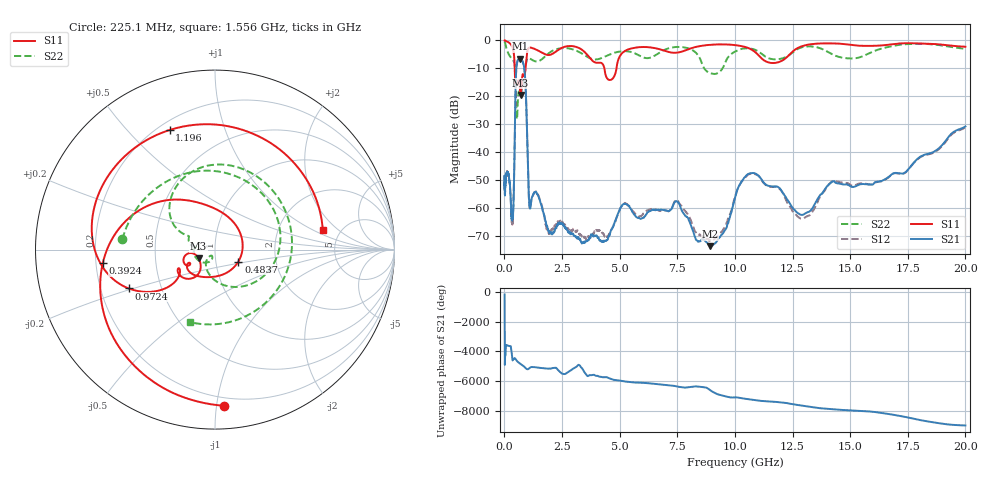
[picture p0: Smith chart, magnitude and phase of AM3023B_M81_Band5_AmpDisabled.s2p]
!Agilent Technologies,E8364B,MY43040894,A.07.50.67
!Agilent E8364B: A.07.50.67
!Date: Tuesday, October 27, 2020 10:38:44
!Correction: S11(Full 2 Port(1,2))
!S21(Full 2 Port(1,2))
!S12(Full 2 Port(1,2))
!S22(Full 2 Port(1,2))
!S2P File: Measurements: S11, S21, S12, S22:Log Frequency Sweep
# Hz S  dB  R 50
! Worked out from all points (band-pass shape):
!   3201 points, 10 MHz to 20 GHz, reference 50 ohm
!   highest |S21| = -6.78 dB at 689.1 MHz (marker M1); lowest = -73.7 dB at 8.919 GHz (marker M2)
!   |S21| within 3 dB of the highest: 523.8 MHz to 855.6 MHz (331.8 MHz wide, 48.1 % of centre)
!   lowest |S11| = -19.7 dB at 704 MHz (marker M3), VSWR 1.23, Z = 41.5 - j4.14 ohm
!   |S11| at or under -10 dB: 447.3 MHz to 919.4 MHz (472.2 MHz wide, 69.1 % of centre); 4.332 GHz to 4.868 GHz (536.3 MHz wide, 11.7 % of centre)
!   |S22| runs from -28.4 to -0.7 dB; largest |S21 - S12| = 0.007
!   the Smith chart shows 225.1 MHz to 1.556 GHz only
!   S11 on the Smith chart (normalised r, x): 225.1 MHz: 0.15, -1.05; 392.4 MHz: 0.23, -0.06; 483.7 MHz: 1.29, -0.17; 972.4 MHz: 0.32, -0.19; 1.196 GHz: 0.24, +0.66; 1.556 GHz: 3.65, +1.29
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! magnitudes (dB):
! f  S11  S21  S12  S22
! 10 MHz  -0.3  -50.9  -48.9  -0.7
! 35.55 MHz  -0.4  -52.6  -52.6  -1.2
! 126.1 MHz  -0.7  -47.2  -47.6  -4.0
! 225.1 MHz  -1.2  -50.6  -51.1  -5.7
! 392.4 MHz  -4.0  -59.3  -58.9  -7.5
! 447.2 MHz  -10.0  -36.1  -36.2  -9.1
! 483.7 MHz  -16.7  -17.5  -17.5  -14.1
! 539.5 MHz  -15.0  -8.7  -8.7  -28.3
! 689.1 MHz  -19.2  -6.8  -6.8  -20.1
! 704 MHz  -19.7  -6.8  -6.8  -20.0
! 873.8 MHz  -12.8  -10.9  -11.0  -13.4
! 972.4 MHz  -5.6  -29.3  -29.4  -7.2
! 1.077 GHz  -2.9  -58.0  -58.5  -6.6
! 1.196 GHz  -2.9  -56.2  -56.3  -7.2
! 1.556 GHz  -4.3  -57.9  -57.6  -7.4
! 1.59 GHz  -4.4  -58.6  -58.2  -7.2
! 3.432 GHz  -4.0  -72.5  -70.5  -5.3
! 5.639 GHz  -2.9  -62.5  -61.7  -4.8
! 8.919 GHz  -1.8  -73.7  -71.6  -11.9
! 10.58 GHz  -3.0  -47.9  -48.1  -3.1
! 13.01 GHz  -2.1  -62.2  -63.6  -2.5
! 20 GHz  -2.5  -31.0  -31.3  -3.3
